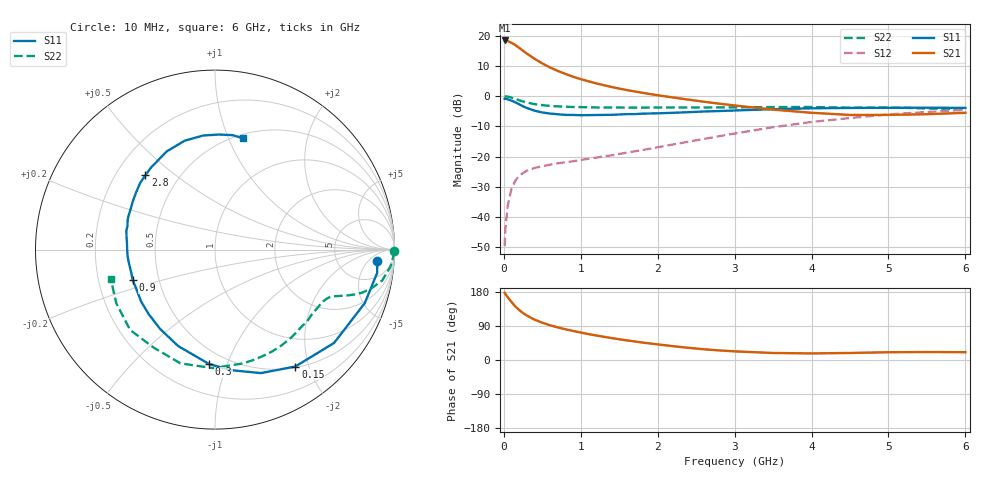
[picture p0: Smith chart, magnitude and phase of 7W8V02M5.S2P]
! Infineon Technologies  Discrete & RF Semiconductors
! BFS17W
! Si NPN RF Bipolar Junction Transistor in SOT323
! VCE = 8 V  IC = 2.5 mA
! Common Emitter S-Parameters:  August  1999
# GHz  S  MA  R  50
!  f  S11  S21  S12  S22
! GHz  MAG  ANG  MAG  ANG  MAG  ANG  MAG  ANG
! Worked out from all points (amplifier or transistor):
!   36 points, 10 MHz to 6 GHz, reference 50 ohm
!   highest |S21| = 18.4 dB at 10 MHz (marker M1)
!   |S21| within 3 dB of that: start of sweep to 228.2 MHz
!   unconditionally stable (mu >= 1): 789.8 MHz to 2.629 GHz; 4.563 GHz to end of sweep
!   at 250 MHz: K = 0.40, MSG = 20.2 dB, |S12| = -25.4 dB
!   at 1.4 GHz: K = 1.25, MAG = 8.3 dB, |S12| = -19.6 dB
!   at 6 GHz: K = 1.07, MAG = -2.1 dB, |S12| = -4.6 dB
!   S11 on the Smith chart (normalised r, x): 10 MHz: 14, -10; 150 MHz: 0.51, -1.79; 300 MHz: 0.40, -0.87; 900 MHz: 0.35, -0.16; 2.8 GHz: 0.32, +0.39; 6 GHz: 0.54, +1.13
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0.01  0.9064 -3.9  8.35 177.6  0.0033 82.3  0.9992 -0.6
0.02  0.9127 -8.2  8.305 174.2  0.0063 89.3  0.994 -2.3
0.05  0.8861 -19.7  8.168 165.7  0.0154 81.5  0.9822 -5.5
0.1  0.843 -38.1  7.627 153.0  0.0296 70.7  0.9479 -10.4
0.15  0.7903 -55.5  6.999 141.2  0.04 62.0  0.8984 -13.9
0.2  0.7341 -69.6  6.294 131.8  0.0485 57.0  0.8548 -16.3
0.25  0.6788 -82.0  5.631 123.8  0.0537 51.8  0.8145 -17.9
0.3  0.6387 -92.9  5.057 117.2  0.0586 49.2  0.7837 -19.0
0.4  0.5753 -110.9  4.149 106.4  0.0649 45.5  0.7378 -20.5
0.5  0.5372 -124.8  3.483 98.4  0.0695 44.5  0.7097 -21.5
0.6  0.5154 -135.9  2.982 91.7  0.0735 44.8  0.6909 -22.6
0.7  0.5028 -145.1  2.622 86.1  0.0773 46.1  0.6786 -23.9
0.9  0.4891 -159.6  2.099 76.6  0.0837 48.7  0.662 -27.0
1.1  0.4855 -171.2  1.762 68.3  0.0922 52.1  0.6544 -30.6
1.3  0.4898 179.3  1.519 61.2  0.1011 55.4  0.6488 -34.7
1.6  0.5051 167.9  1.261 51.7  0.1163 60.5  0.6458 -41.1
2.2  0.5311 149.5  0.952 36.4  0.1589 68.0  0.6498 -55.6
2.8  0.5674 133.2  0.752 25.3  0.2176 70.2  0.6514 -71.5
3.5  0.6096 116.2  0.6 18.5  0.3065 67.6  0.6606 -91.0
4.5  0.639 95.9  0.489 18.5  0.4344 55.9  0.6442 -122.2
5.5  0.6451 81.4  0.503 21.0  0.5478 42.4  0.6259 -151.5
6  0.6399 75.9  0.531 20.6  0.5922 35.8  0.6033 -164.5
